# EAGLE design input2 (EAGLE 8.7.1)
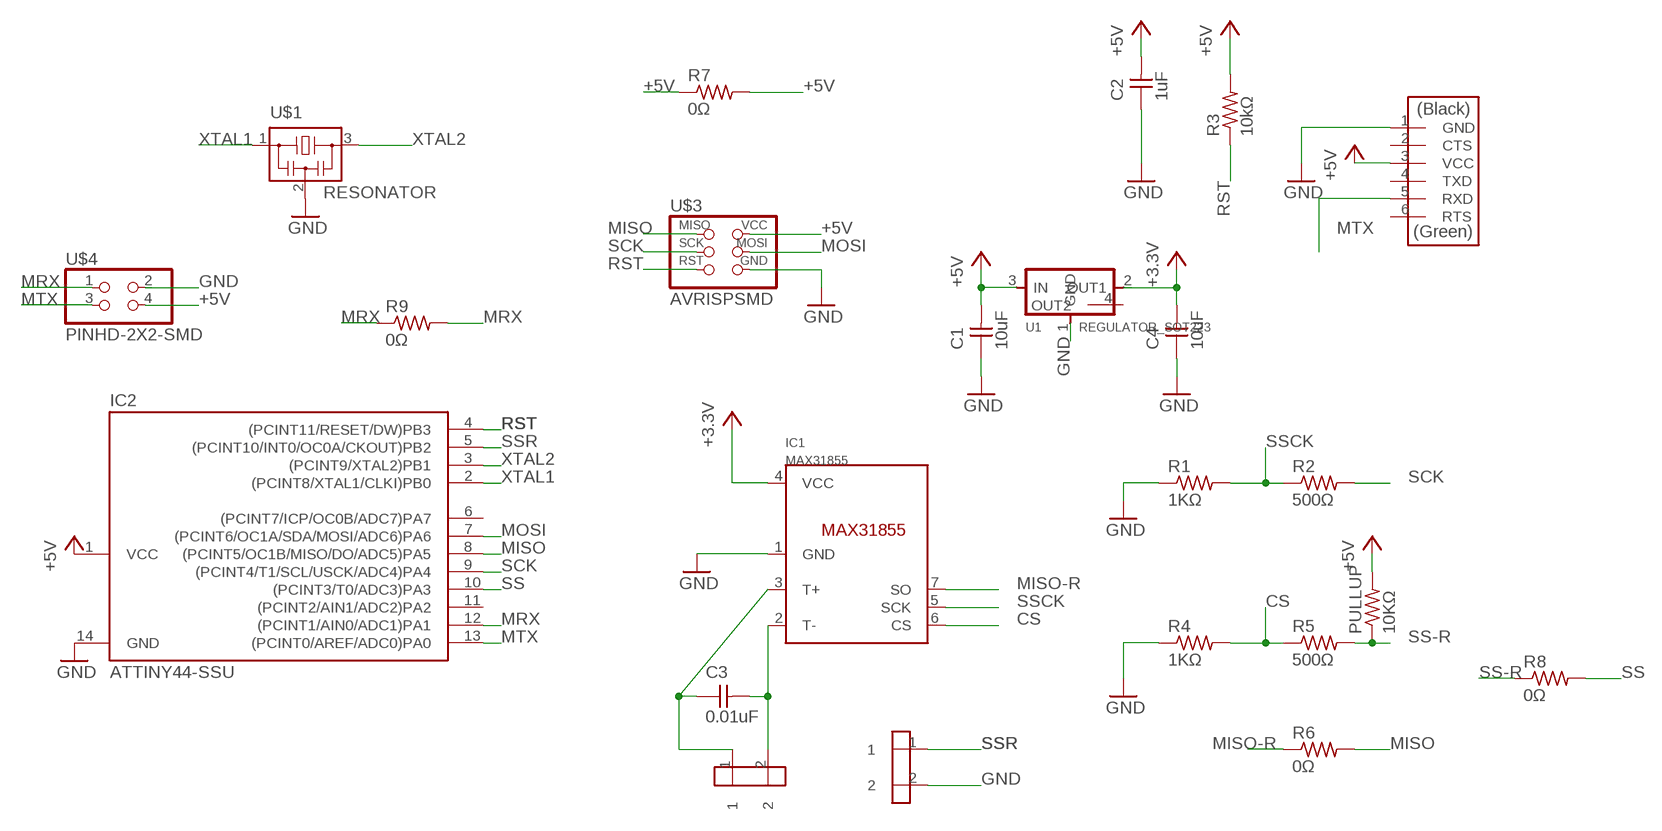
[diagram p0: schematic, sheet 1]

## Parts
C1  10uF  CAP-UNPOLARIZEDFAB  [C1206FAB]
C2  1uF  CAP-UNPOLARIZED  [C1206]
C3  0.01uF  CAP-UNPOLARIZEDFAB  [C1206FAB]
C4  10uF  CAP-UNPOLARIZEDFAB  [C1206FAB]
IC1  MAX31855  [SOIC8]
IC2  ATTINY44-SSU  [SOIC14]
PULLUP  10KΩ  RES-US1206FAB  [R1206FAB]
R1  1KΩ  RES-US1206FAB  [R1206FAB]
R2  500Ω  RES-US1206FAB  [R1206FAB]
R3  10kΩ  RES-US1206  [R1206]
R4  1KΩ  RES-US1206FAB  [R1206FAB]
R5  500Ω  RES-US1206FAB  [R1206FAB]
R6  0Ω  RES-US1206FAB  [R1206FAB]
R7  0Ω  RES-US1206FAB  [R1206FAB]
R8  0Ω  RES-US1206FAB  [R1206FAB]
R9  0Ω  RES-US1206FAB  [R1206FAB]
SSR  AKIZUKITNK_HOLE2PIN  [5.08PICH_HL]
TML1  AKIZUKITNK_HOLE2PIN  [5.08PICH_HL]
U1  REGULATOR_SOT223  [SOT223]
U$1  RESONATOR  [EFOBM]
U$2  FTDI-SMD-HEADER  [1X06SMD]
U$3  AVRISPSMD  [2X03SMD]
U$4  PINHD-2X2-SMD  [2X02SMD]

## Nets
3.3V: C4.2 IC1.4(VCC) U1.2(OUT1) ; supply symbol labelled +3.3V
+5V: C1.2 C2.2 IC2.1(VCC) PULLUP.2 R3.2 R7.1 R7.2 U1.3(IN) U$2.3(VCC) U$3.2(VCC) U$4.4
CS: IC1.6(CS) R4.2 R5.1
GND: C1.1 C2.1 C4.1 IC1.1(GND) IC2.14(GND) R1.1 R4.1 SSR.2 U1.1(GND) U$1.2 U$2.1(GND) U$3.6(GND) U$4.2
MISO: IC2.8((PCINT5/OC1B/MISO/DO/ADC5)PA5) R6.2 U$3.1(MISO)
MISO-R: IC1.7(SO) R6.1
MOSI: IC2.7((PCINT6/OC1A/SDA/MOSI/ADC6)PA6) U$3.4(MOSI)
MRX: IC2.12((PCINT1/AIN0/ADC1)PA1) R9.1 R9.2 U$4.1
MTX: IC2.13((PCINT0/AREF/ADC0)PA0) U$2.5(RXD) U$4.3
N$2: C3.1 IC1.3(T+) TML1.1
N$3: C3.2 IC1.2(T-) TML1.2
RST: IC2.4((PCINT11/RESET/DW)PB3) R3.1 U$3.5(RST)
SCK: IC2.9((PCINT4/T1/SCL/USCK/ADC4)PA4) R2.2 U$3.3(SCK)
SS: IC2.10((PCINT3/T0/ADC3)PA3) R8.2
SS-R: PULLUP.1 R5.2 R8.1
SSCK: IC1.5(SCK) R1.2 R2.1
SSR: IC2.5((PCINT10/INT0/OC0A/CKOUT)PB2) SSR.1
XTAL1: IC2.2((PCINT8/XTAL1/CLKI)PB0) U$1.1
XTAL2: IC2.3((PCINT9/XTAL2)PB1) U$1.3
Unconnected: IC2.6((PCINT7/ICP/OC0B/ADC7)PA7) IC2.11((PCINT2/AIN1/ADC2)PA2) U1.4(OUT2) U$2.2(CTS) U$2.4(TXD) U$2.6(RTS)

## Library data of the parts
C1-C4 = fab:CAP-UNPOLARIZED
IC1 = AlexW-Eagle-Libraries 2:MAX31855
IC2 = fab:ATTINY44
PULLUP R1 R2 R4-R6 R8 = fab:RES-US: Resistor (US Symbol)
R3 R7 R9 = HelloKamakura:RES-US: Resistor (US Symbol)
SSR TML1 = doyo:AKIZUKI?TNK_HOLE2PIN
U1 = fab:REGULATOR_SOT223
U$1 = fab:RESONATOR
U$2 = fab:FTDI-SMD-HEADER
U$3 = HelloKamakura:AVRISP
U$4 = fab:PINHD-2X2-SMD

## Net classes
0 default: width 0.406 mm

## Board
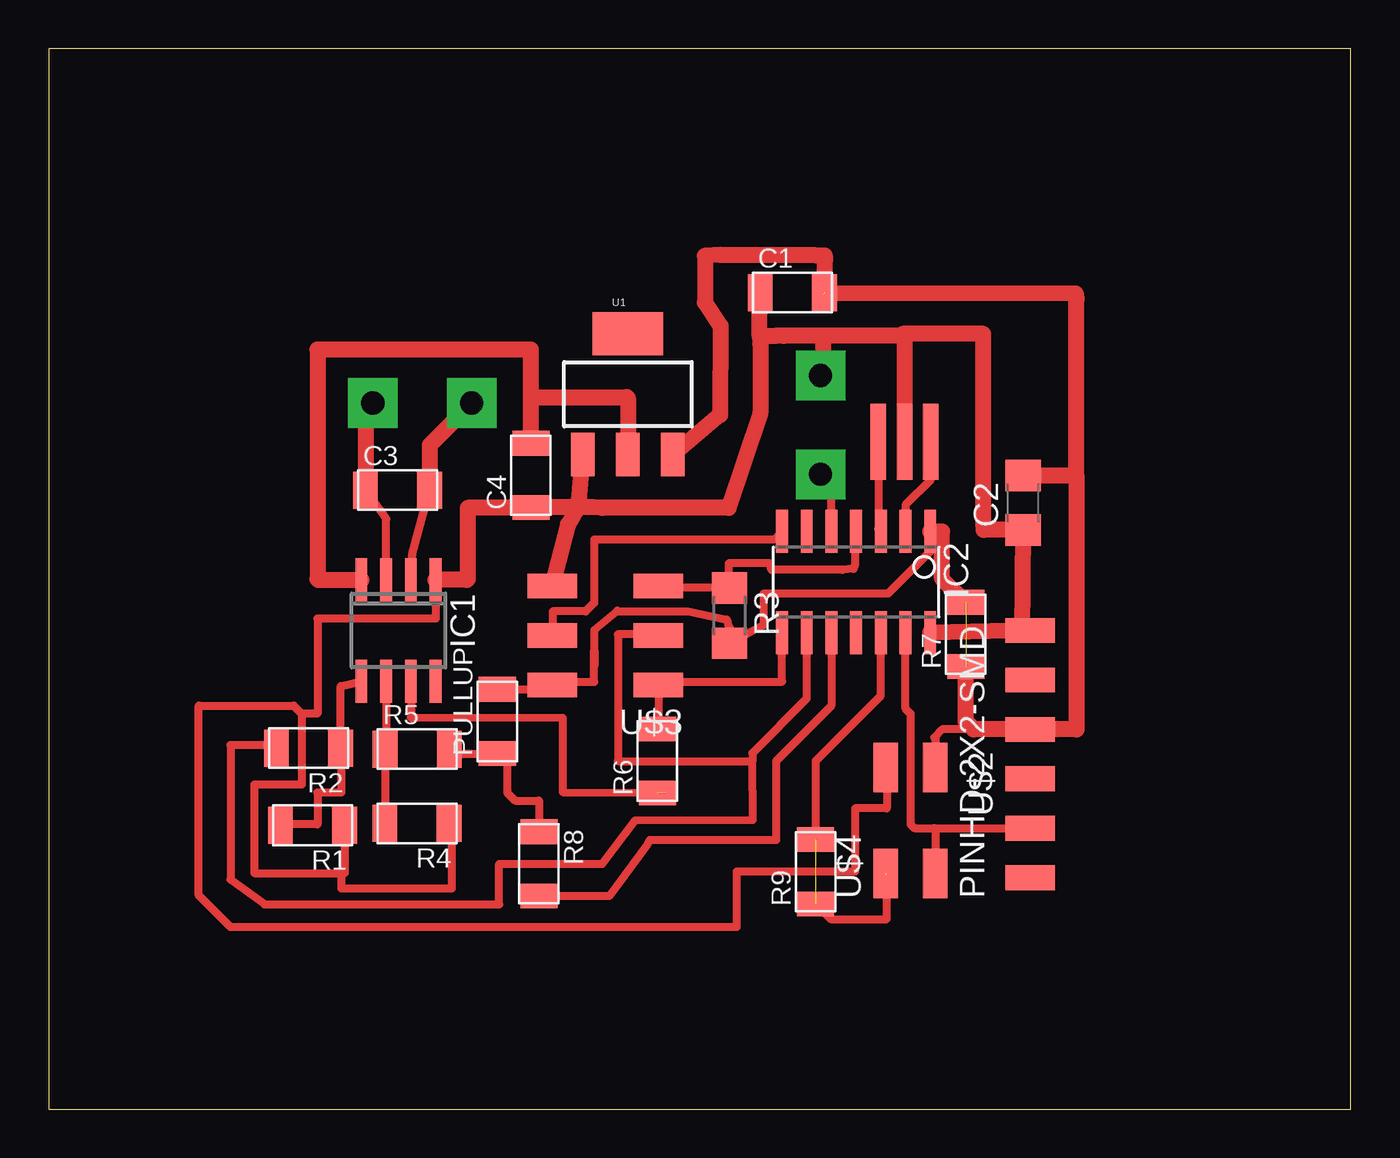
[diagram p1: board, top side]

Size 66.93 x 54.48 mm. Coordinates in mm from the lower left corner, seen from the top.
Outline: 0,0 66.93,0 66.93,54.48 0,54.48 0,0
Copper layers (1*16): Top 0.035mm / dielectric 1.5mm / Bottom 0.035mm
Design rules "default *": minimum track width 6mil, minimum drill 0.35mm, track to track 0.4mm, track to pad 0.4mm, pad to pad 0.4mm, via to via 0.4mm, smd to smd 0.4mm, copper to edge 40mil, drill to drill 6mil, minimum pad ring 10mil, minimum via ring 8mil, stop-mask expansion 4mil, vias tented up to drill 0mil, thermal gap 10mil

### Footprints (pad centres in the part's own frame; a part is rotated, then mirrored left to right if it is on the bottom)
C1206FAB = smd 1.27 x 1.905: 1 -1.651,0; 2 1.651,0
C1206 = smd 1.6 x 1.8: 1 -1.4,0; 2 1.4,0
SOIC8 = smd 0.6 x 2.2: 1 -1.905,-2.6; 2 -0.635,-2.6; 3 0.635,-2.6; 4 1.905,-2.6; 5 1.905,2.6; 6 0.635,2.6; 7 -0.635,2.6; 8 -1.905,2.6
SOIC14 = smd 0.61 x 2.21: 1 -3.81,-2.603; 2 -2.54,-2.603; 3 -1.27,-2.603; 4 0,-2.603; 5 1.27,-2.603; 6 2.54,-2.603; 7 3.81,-2.603; 8 3.81,2.603; 9 2.54,2.603; 10 1.27,2.603; 11 0,2.603; 12 -1.27,2.603; 13 -2.54,2.603; 14 -3.81,2.603
R1206FAB = smd 1.27 x 1.905: 1 -1.651,0; 2 1.651,0
R1206 = smd 1.6 x 1.803: 1 -1.422,0; 2 1.422,0
5.08PICH_HL = drill 1.2 pad 2.54 square: 1 0,0; 2 -5.08,0
SOT223 = smd 1.219 x 2.235: 1 -2.311,-3.099; 2 0,-3.099; 3 2.311,-3.099 | smd 3.6 x 2.2: 4 0,3.099
EFOBM = smd 0.8 x 3.9: 1 -1.35,0; 2 0,0; 3 1.35,0
1X06SMD = smd 2.54 x 1.27: 1 0,6.35; 2 0,3.81; 3 0,1.27; 4 0,-1.27; 5 0,-3.81; 6 0,-6.35
2X03SMD = smd 2.54 x 1.27: 1 -2.54,2.54; 2 2.92,2.54; 3 -2.54,0; 4 2.92,0; 5 -2.54,-2.54; 6 2.92,-2.54
2X02SMD = smd 2.54 x 1.27: 1 -2.54,1.27; 2 2.92,1.27; 3 -2.54,-1.27; 4 2.92,-1.27

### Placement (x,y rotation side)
C1  38.23,41.95 0 top
C2  50.09,31.15 90 top
C3  17.93,31.8 0 top
C4  24.79,32.56 90 top
IC1  17.98,24.59 180 top
IC2  41.5,27.08 180 top
PULLUP  23.06,19.91 90 top
R1  13.56,14.58 180 top
R2  13.36,18.54 180 top
R3  35,25.35 270 top
R4  18.94,14.68 180 top
R5  18.95,18.49 0 top
R6  31.29,17.88 90 top
R7  47.14,24.38 90 top
R8  25.2,12.6 270 top
R9  39.42,12.19 90 top
SSR  39.67,32.61 270 top
TML1  16.66,36.27 180 top
U1  29.77,36.73 0 top
U$1  43.99,34.29 180 top
U$2  50.44,18.24 0 top
U$3  28.8,24.33 180 top
U$4  44.3,14.63 90 top

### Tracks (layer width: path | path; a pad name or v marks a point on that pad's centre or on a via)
3.3V
  Top 0.813: C4.2 24.79,36.58 | 24.79,36.58 29.72,36.58 29.77,36.52 U1.2 | 24.79,36.58 24.79,39.01 13.82,39.01 13.82,27.23 13.86,27.19 IC1.4
+5V  (2 unrouted)
  Top 0.406: 28.04,22.76 28.04,21.95 26.04,21.95 U$3.2 25.88,21.57 PULLUP.2 | 28.04,22.76 28.04,23.57 28.05,23.58 | 28.05,23.58 28.05,22.77 28.04,22.76 | 28.05,23.58 28.05,24.62 29.23,25.6 29.29,25.57 32.86,25.57 34.86,25.15 34.95,24.79 35,24.74 R3.2 36.75,24.87 36.75,26.48 43.14,26.48 45.31,28.65 45.31,29.67 IC2.1 | 47.55,19.51 45.92,19.51 45.52,19.1 45.57,19.05 U$4.4
  Top 0.813: 50.76,32.66 49.98,32.55 C2.2 52.79,32.55 52.83,32.51 | 39.45,43.87 34.54,43.89 | 34.54,43.89 33.73,43.84 33.73,41.45 34.54,40.23 34.52,35.66 U1.3 | 34.54,43.89 39.89,43.87 39.83,41.86 | 52.83,32.51 52.83,41.59 52.79,41.91 C1.2 | 52.83,32.51 52.83,19.51 U$2.3 47.55,19.51 47.14,19.91 R7.1 | R7.2 45.92,27.25 45.92,29.67 45.31,29.67
CS
  Top 0.406: R4.2 17.3,14.68 17.3,18.29 | R5.1 17.3,18.29 | 17.35,18.29 17.3,18.29 | IC1.6 17.35,18.34 17.3,18.29
GND
  Top 0.406: 20.57,14.67 R4.1 20.73,14.68 20.73,11.34 15.04,11.34 15.04,12.12 | IC1.1 19.89,25.22 19.91,25.2 13.82,25.2 13.82,20.32 13.01,20.32 | 13.01,20.32 13.01,16.66 10.57,16.66 10.57,12.12 15.04,12.12 | R1.1 15.21,12.12 15.04,12.12 | U$4.2 43.08,17.5 43.08,15.44 41.45,15.44 41.45,12.19 35.36,12.19 35.36,9.35 9.35,9.35 7.72,10.97 7.72,20.73 12.6,20.73 13.01,20.32
  Top 0.813: IC2.14 U$2.1 50.02,24.43 C2.1 48.06,29.75 48.04,30.07 48.04,39.83 43.89,39.83 43.99,39.73 | 43.99,39.73 U$1.2 | 43.99,39.73 39.83,39.73 | 39.83,39.73 37.8,39.73 | 37.8,39.73 37.34,39.73 36.58,39.71 | 37.8,39.73 36.54,39.71 | 36.54,39.71 36.55,39.67 36.58,39.32 36.58,35.76 34.95,30.89 28.45,30.89 | 28.45,30.89 27.23,30.96 | 27.23,30.96 U1.1 | 28.45,30.89 27.2,30.91 C4.1 24.36,30.89 21.54,30.89 21.54,27.23 21.5,27.19 IC1.1 | 27.23,30.96 26.7,30.02 U$3.6 | SSR.2 39.83,37.85 39.83,39.73 | 36.54,39.71 36.54,41.98 C1.1
MISO
  Top 0.406: IC2.8 37.69,21.97 37.68,21.96 31.51,21.96 U$3.1 31.34,19.58 R6.2
MISO-R  (1 unrouted)
  Top 0.406: IC1.7 18.62,20.13 18.68,20.07 18.69,20.07 26.42,20.09 26.42,16.28 31.7,16.26
MOSI
  Top 0.406: IC2.7 37.27,29.26 28.04,29.26 28.04,26.01 27.6,25.57 25.91,25.57 25.91,24.36 U$3.4
MRX  (2 unrouted)
  Top 0.406: R9.1 40.21,9.75 43.08,9.75 43.08,12.04 | R9.2 39.42,17.88 42.77,21.23 IC2.12
MTX
  Top 0.406: 45.52,14.43 44.5,14.43 44.3,14.63 44.3,20.32 44.04,20.57 IC2.13 | 45.52,14.43 45.57,14.38 U$4.3 | 45.52,14.43 U$2.5
N$2
  Top 0.406: IC1.3 17.35,30.33 C3.1
  Top 0.813: TML1.1 16.28,35.89 C3.1
N$3
  Top 0.406: IC1.2 18.69,27.26 18.69,28.47 C3.2
  Top 0.813: TML1.2 19.58,34.11 C3.2
RST
  Top 0.406: IC2.4 41.45,29.63 41.44,27.91 41.38,27.75 40.81,27.7 37.16,27.7 37.07,28.04 34.95,28.04 34.95,26.82 | 34.95,26.82 R3.1 | U$3.5 31.39,26.82 34.95,26.82
SCK
  Top 0.406: U$3.3 31.29,24.38 29.26,24.38 29.26,17.88 36.17,17.88 | 39.01,24.42 IC2.9 38.96,21.08 36.17,18.29 36.17,17.88 | R2.2 11.56,18.69 9.35,18.69 9.35,11.79 11.1,10.52 23.16,10.52 23.16,12.6 28.45,12.6 30.15,14.83 36.2,14.86 36.17,17.88
SS
  Top 0.406: R8.2 28.83,10.95 30.79,13.61 30.89,13.82 37.39,13.82 37.39,17.88 40.23,20.73 IC2.10
SS-R
  Top 0.406: 23.06,18.49 PULLUP.1 | R5.2 20.83,18.26 PULLUP.1 | PULLUP.1 23.57,17.75 23.57,16.26 23.98,15.85 25.2,15.85 R8.1
SSCK
  Top 0.406: R2.1 15.01,21.73 IC1.5 | 15.04,18.69 14.86,18.69 R2.1 | R2.1 15.04,18.54 15.04,16.26 13.82,16.26 13.82,14.63 11.91,14.63 R1.2
SSR
  Top 0.406: IC2.5 40.23,32.05 SSR.1
XTAL1
  Top 0.406: U$1.1 45.34,32.34 44.04,31.04 IC2.2
XTAL2
  Top 0.406: U$1.3 42.64,29.81 IC2.3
